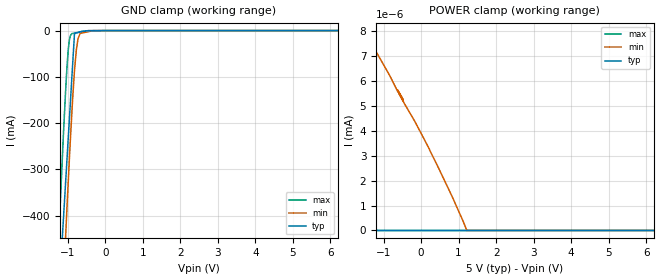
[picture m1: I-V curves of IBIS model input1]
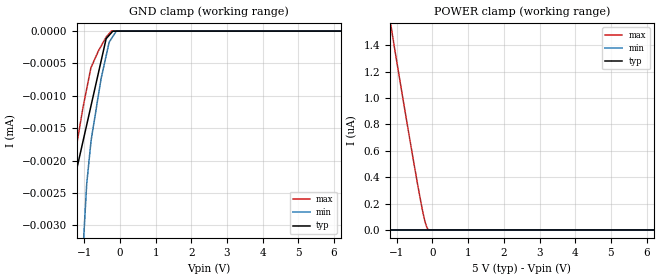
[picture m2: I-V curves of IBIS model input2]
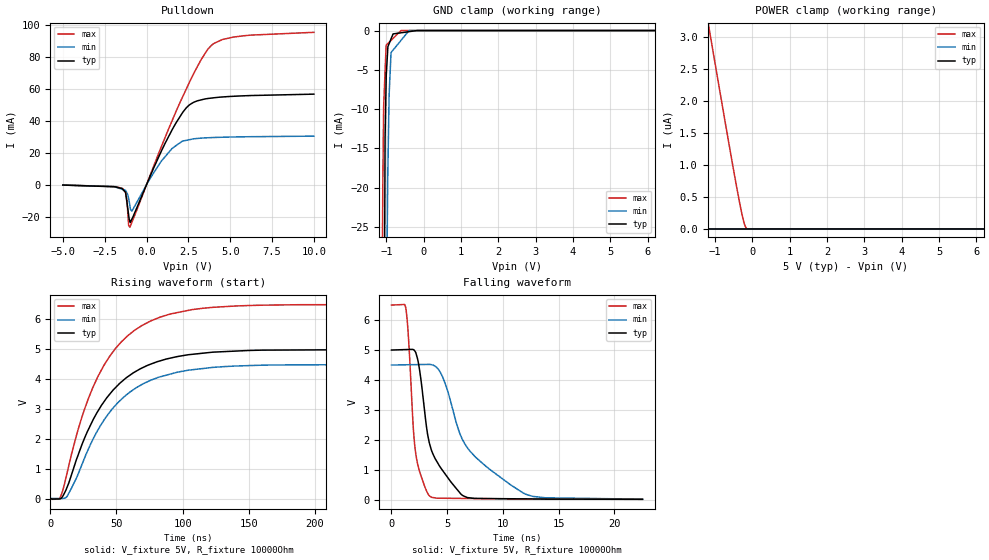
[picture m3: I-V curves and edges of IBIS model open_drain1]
| Texas Instruments Incorporated
| TPS2547 USB Charging Port Controller and 3-Amp Power Switch With Load
| Detection
[IBIS Ver]   4.1
[File name]   tps2547.ibs
[File Rev]   1.0
[Date]   02/07/2018
[Source]
| Texas Instruments Incorporated.
| Analog-eLab Design Center, HPA
| 12500 TI Blvd
| Dallas, TX -75243
[Notes]   Revision History:
| Rev 1.0: 02/07/2018
| - Initial version of the model
| - Model generated from simulations in SPECTRE
| - C_comp although listed in numerical order of value are
|   obtained from varying PVT conditions. For PVT conditions for
|   each specific value refer the buffer description under
|   respective [Model]. IBIS model user is responsible for using
|   appropriate C_comp to simulate for Signal Integrity.
| - Warnings regarding combined Non-monotonicity of various models
|   have been reviewed and considered minor and can be ignored.
[Disclaimer]
| This model is designed as an aid for customers of Texas Instruments.
| TI and its licensors and suppliers make no warranties, either expressed
| or implied, with respect to this  model, including the warranties of
| merchantability or fitness for a particular purpose. The model is
| provided solely on an "as is" basis. The entire risk as to its quality
| and performance is with the customer.
| This model is subject to change without notice. Texas Instruments
| Incorporated is not responsible for updating this model.
[Copyright]
(C) Copyright 2018 Texas Instruments Incorporated.All rights reserved.
|  Component TPS2547 16-pin WQFN - RTE Package
|  Part # TPS2547
[Component]   TPS2547
[Manufacturer]   TI
[Package]   |16 WQFN - RTE Package
|   typ   min   max
R_pkg   0.1   0.08   0.12
L_pkg   1.0nH   0.8nH   1.2nH
C_pkg   0.2pF   0.16pF   0.24pF
[Pin]   signal_name   model_name   R_pin   L_pin   C_pin
1   IN   power   NA   NA   NA
2   DM_OUT   nc   NA   NA   NA
3   DP_OUT   nc   NA   NA   NA
4   ILIM_SEL   nc   NA   NA   NA
5   EN   input2   NA   NA   NA
6   CTL1   input1   NA   NA   NA
7   CTL2   input1   NA   NA   NA
8   CTL3   input1   NA   NA   NA
9   _STATUS   open_drain2   NA   NA   NA
10   DP_IN   nc   NA   NA   NA
11   DM_IN   nc   NA   NA   NA
12   OUT   power   NA   NA   NA
13   _FAULT   open_drain1   NA   NA   NA
14   GND   gnd   NA   NA   NA
15   ILIM_LO   nc   NA   NA   NA
16   ILIM_HI   nc   NA   NA   NA
| Models and submodels in the file (4): input1 (Input), input2 (Input), open_drain1 (Open_drain), open_drain2 (Open_drain)
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|   input1 Model
[Model]   input1
Model_type   Input
Vinl = 1.15
Vinh = 1.35
|   typ   min   max
C_comp   0.3923pF   0.3645pF   0.4309pF
|  Where Nom  PVT is Nominal Process,   5V,  27C
|   Fast PVT is Strong Process,   6.5V, -40C
|   Slow PVT is Weak Process,   4.5V, 125C
[Model spec]
|subparameter
[Voltage Range]   5   4.5   6.5
|Junction Temperature
[Temperature Range]   27   125   -40
[Power Clamp Reference]   5   4.5   6.5
[GND Clamp Reference]   0   0   0
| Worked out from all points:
|   GND clamp passes 1 mA (typ) near -0.54 V on its own axis
|   POWER clamp passes 1 mA (typ) near -3.63 V on its own axis
[GND Clamp]
|   Voltage   I(typ)   I(min)   I(max)
-5V       -7.959A    -8.135A    -7.854A
-1.25V    -593.5mA   -794.9mA   -467.6mA
-1.123V   -421.1mA   -565mA     -242.5mA
-1.059V   -333.5mA   -452.8mA   -136.5mA
-1.034V   -300.7mA   -410.7mA   -101.2mA
-987.5mV  -236.8mA   -332.3mA   -44.55mA
-959.3mV  -198.5mA   -286.2mA   -22.86mA
-890.3mV  -104.6mA   -181mA     -6.456mA
-818.7mV  -7.303mA   -87.43mA   -5.416mA
-723.1mV  -3.918mA   -17.61mA   -4.024mA
-314.9mV  -586.4uA   -42.46uA   -3.11uA
10V       0A         0A         0A
[POWER Clamp]
|   Voltage   I(typ)   I(min)   I(max)
-5V       223.5mA    118.7mA    505.5mA
-2.067V   8.804uA    4.489uA    236.3uA
-1.25V    0A         7.927nA    2.104nA
-1.25V    0A         7.887nA    0A
-1.25V    0A         7.318nA    0A
-497.2mV  0A         5.315nA    0A
-482.5mV  0A         5.196nA    0A
-482.3mV  0A         5.275nA    0A
225.8mV   0A         3.253nA    0A
842.8mV   0A         1.314nA    0A
1.219V    0A         0A         0A
10V       0A         0A         0A
|   input2 Model
[Model]   input2
Model_type   Input
Vinl = 1.15
Vinh = 1.35
|   typ   min   max
C_comp   0.2196pF   0.2021pF   0.2353pF
|  Where Nom  PVT is Nominal Process,   5V,  27C
|   Fast PVT is Strong Process,   6.5V, -40C
|   Slow PVT is Weak Process,   4.5V, 125C
[Model spec]
|subparameter
[Voltage Range]   5   4.5   6.5
|Junction Temperature
[Temperature Range]   27   125   -40
[Power Clamp Reference]   5   4.5   6.5
[GND Clamp Reference]   0   0   0
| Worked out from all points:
|   GND clamp passes 1 mA (typ) near -1.95 V on its own axis
[GND Clamp]
|   Voltage   I(typ)   I(min)   I(max)
-5V       -446.6mA   -497.4mA   -405.2mA
-1.905V   -930.2uA   -4.269mA   -308.2uA
-1.25V    -2.23uA    -12.84uA   -1.892uA
-1.018V   -1.662uA   -3.222uA   -1.135uA
-930.2mV  -1.448uA   -2.363uA   -892.4nA
-809mV    -1.152uA   -1.696uA   -564.1nA
-530.1mV  -470.6nA   -742.9nA   -235.3nA
-385.9mV  -118nA     -382.7nA   -93.68nA
-301.5mV  -65.24nA   -172.1nA   -39.3nA
-240.6mV  -27.17nA   -119.8nA   -34.01pA
-100.8mV  -514.1pA   -3.663pA   0A
10V       0A         0A         0A
[POWER Clamp]
|   Voltage   I(typ)   I(min)   I(max)
-5V       8.152uA    7.795uA    12.6uA
-2.614V   1.977uA    1.712uA    5.238uA
-2.435V   1.624uA    1.379uA    4.737uA
-2.366V   1.517uA    1.252uA    4.546uA
-1.703V   503.1nA    211.7nA    2.715uA
-1.512V   230.6nA    20.97nA    2.249uA
-1.25V    0A         2.67pA     1.703uA
-1.119V   0A         0A         1.474uA
-386mV    0A         0A         300.5nA
-229.8mV  0A         0A         86.15nA
-119.4mV  0A         0A         41.9pA
10V       0A         0A         0A
|   open_drain1 Model
[Model]   open_drain1
Model_type   Open_drain
Polarity   Non-Inverting
Vmeas = 2.5
Vref = 5
Cref = 10pF
Rref = 10000
|   typ   min   max
C_comp   0.4015pF   0.3834pF   0.4362pF
|  Where Nom  PVT is Nominal Process,   5V,  27C
|   Fast PVT is Strong Process,   6.5V, -40C
|   Slow PVT is Weak Process,   4.5V, 125C
[Voltage Range]   5   4.5   6.5
|Junction Temperature
[Temperature Range]   27   125   -40
[Pullup Reference]   5   4.5   6.5
[Pulldown Reference]   0   0   0
[Power Clamp Reference]   5   4.5   6.5
[GND Clamp Reference]   0   0   0
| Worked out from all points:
|   slope of the pulldown table from 0 to 0.75 V, typ, clamps not added: 41.9 ohm
|   GND clamp passes 1 mA (typ) near -0.87 V on its own axis
|   falling waveform, V_fixture 5V, R_fixture 10000Ohm: 20-80 % time 1.88ns typ, 4.12ns min, 721ps max; typ from 5 V to 0.02 V
|   rising waveform, V_fixture 5V, R_fixture 10000Ohm: 20-80 % time 38.6ns typ, 39.3ns min, 37.7ns max; typ from 0.02 V to 5 V
[Pulldown]
|   Voltage   I(typ)   I(min)   I(max)
-5V       -197.6uA   -199.9uA   -158.6uA
-1.431V   -2.702mA   -2.897mA   -2.362mA
-1.25V    -4.745mA   -3.497mA   -5.035mA
-1.163V   -11.55mA   -5.304mA   -10.43mA
-1.067V   -19.02mA   -8.768mA   -25.61mA
-993.5mV  -22.92mA   -13.06mA   -26.56mA
-870.9mV  -21.44mA   -16.46mA   -23.41mA
1.75V     38.51mA    24.41mA    45.52mA
2.569V    50.07mA    28.23mA    64.28mA
3.671V    54.03mA    29.43mA    85mA
5.178V    55.4mA     29.91mA    92.45mA
10V       56.74mA    30.44mA    95.46mA
[GND Clamp]
|   Voltage   I(typ)   I(min)   I(max)
-5V       -7.609A    -7.671A    -7.581A
-1.118V   -116.2mA   -170.7mA   -36.35mA
-1.097V   -89.24mA   -141.1mA   -19.9mA
-1.074V   -61.13mA   -111.5mA   -9.713mA
-1.038V   -16.37mA   -70.49mA   -5.474mA
-1.036V   -13.65mA   -68.23mA   -5.205mA
-1.007V   -6.423mA   -44.03mA   -1.867mA
-966.1mV  -2.54mA    -19.43mA   -1.676mA
-927.3mV  -1.67mA    -8.186mA   -1.494mA
-875.5mV  -1.066mA   -2.806mA   -1.253mA
-607.2mV  -290uA     -1.247mA   0A
10V       0A         0A         0A
[POWER Clamp]
|   Voltage   I(typ)   I(min)   I(max)
-5V       11.65uA    11.71uA    16.49uA
-2.827V   4.514uA    4.035uA    8.906uA
-2.263V   2.685uA    2.089uA    6.952uA
-1.698V   912.6nA    300.5nA    4.998uA
-1.579V   553.8nA    60.33nA    4.586uA
-1.491V   319.8nA    25.32pA    4.279uA
-1.386V   76.36nA    14.35pA    3.917uA
-1.25V    0A         0A         3.444uA
-1.036V   0A         0A         2.711uA
-341.7mV  0A         0A         409.6nA
-144.6mV  0A         0A         0A
10V       0A         0A         0A
[Ramp]
R_load = 10000
|   typ   min   max
dV/dt_r   2.98809/3.86482e-08   2.68559/3.93281e-08   3.88591/3.77127e-08
dV/dt_f   2.98809/1.8726e-09   2.68559/4.10169e-09   3.88591/7.20645e-10
[Falling Waveform]
V_fixture = 5V
V_fixture_min = 4.5V
V_fixture_max = 6.5V
R_fixture = 10000Ohm
C_fixture = 0F
|   Time   V(typ)   V(min)   V(max)
0s        5V         4.5V       6.5V
1.272ns   5.015V     4.508V     6.421V
1.488ns   5.018V     4.509V     5.608V
1.931ns   5.018V     4.512V     2.55V
2.152ns   4.933V     4.513V     1.609V
3.414ns   1.875V     4.52V      132.4mV
4.604ns   972.1mV    4.088V     56.09mV
6.414ns   140.2mV    1.98V      49.7mV
11.79ns   35.1mV     235.3mV    30.73mV
22.52ns   19.84mV    24.02mV    23.42mV
[Rising Waveform]
V_fixture = 5V
V_fixture_min = 4.5V
V_fixture_max = 6.5V
R_fixture = 10000Ohm
C_fixture = 0F
|   Time   V(typ)   V(min)   V(max)
0s        19.84mV    24.01mV    23.42mV
8.275ns   29.25mV    22.65mV    142.5mV
12.91ns   422.9mV    108.5mV    916.4mV
23.63ns   1.788V     1.123V     2.704V
40.4ns    3.241V     2.628V     4.458V
53.82ns   3.919V     3.339V     5.259V
75.74ns   4.507V     3.968V     5.948V
107ns     4.836V     4.32V      6.328V
140.2ns   4.945V     4.446V     6.451V
300ns     5V         4.5V       6.5V
